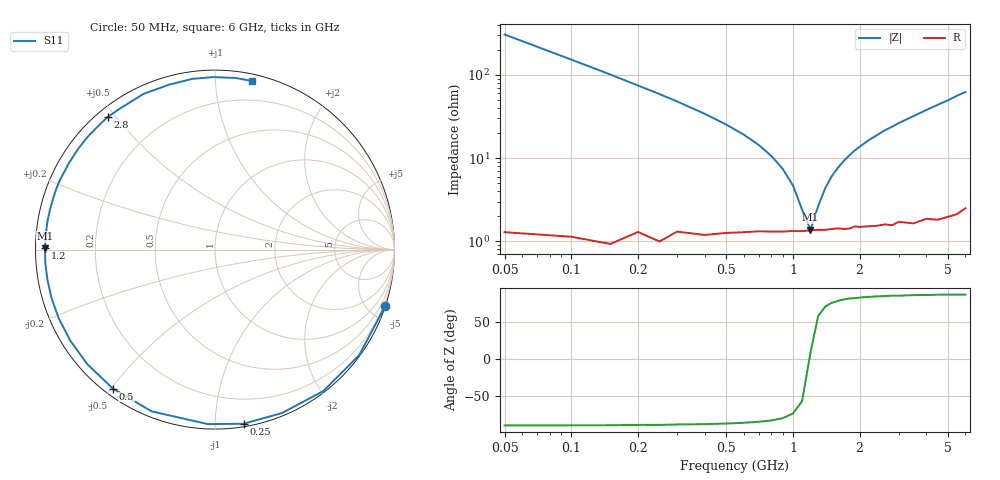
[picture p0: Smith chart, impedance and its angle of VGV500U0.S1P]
! Infineon Technologies  Discrete & RF Semiconductors
! BB 831
! Si Tuning Diode in SOD323
! VR = 0.5 V
! S-Parameters:  July  1999
# GHz  S  MA  R  50
!  f  S11
! GHz  MAG  ANG
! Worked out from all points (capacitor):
!   34 points, 50 MHz to 6 GHz, reference 50 ohm
!   read as one part to ground: C = 10.3 pF near 50 MHz
!   lowest |Z| = 1.38 ohm at 1.2 GHz (marker M1)
!   series resonance near 1.19 GHz, so ESL is about 1.7 nH
!   S11 on the Smith chart (normalised r, x): 50 MHz: 0.03, -6.14; 250 MHz: 0.02, -1.18; 500 MHz: 0.03, -0.51; 1.2 GHz: 0.03, +0.00; 2.8 GHz: 0.03, +0.48; 6 GHz: 0.05, +1.24
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0.05  0.9987 -18.5
0.1  0.9956 -36.2
0.15  0.9928 -52.5
0.2  0.9841 -67.6
0.25  0.9835 -80.6
0.3  0.9732 -92.3
0.4  0.968 -111.4
0.5  0.9606 -126.3
0.6  0.9561 -138.1
0.7  0.9524 -147.9
0.8  0.9511 -156.2
0.9  0.95 -163.4
1  0.9486 -169.7
1.2  0.9471 179.5
1.4  0.9468 170.5
1.6  0.9457 162.7
1.9  0.9446 152.4
2.2  0.9467 143.6
2.4  0.9476 138.5
2.6  0.9476 133.3
2.8  0.9504 129.0
3  0.9477 124.4
3.5  0.9545 114.7
4  0.9538 105.6
4.5  0.9597 97.5
5  0.9611 90.5
5.5  0.9633 83.2
6  0.9616 77.5
